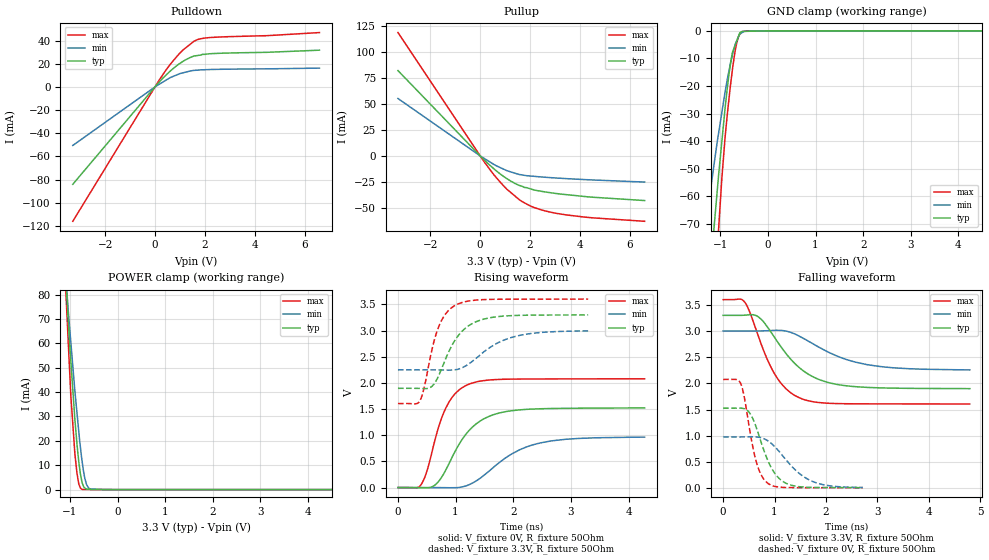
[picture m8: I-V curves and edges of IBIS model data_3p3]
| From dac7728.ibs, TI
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|   data_3p3 Model
[Model]   data_3p3
Model_type   I/O
Polarity   Non-Inverting
Enable   Active-Low
Vinl = 0.6
Vinh = 2.3
Vmeas = 1.65
Vref = 1.65
Cref = 10pF
Rref = 50
|   typ   min   max
|   (nom PVT)   (Fast PVT)   (slow PVT)
|C_comp from frequency method(F=50MHz)
|Average
C_comp   9.480e-12   7.960e-12   1.096e-11
|ON state : BUFFER OUTPUT TURNED HIGH
|C_comp   9.694e-12   8.160e-12   1.122e-11
|OFF state: BUFFER IN HIGH IMPEDANCE
|C_comp   9.266e-12   7.761e-12   1.070e-11
|C_comp from L-C Tank method(L=1nH)
|Average
|C_comp   8.7775e-12  7.5775e-12  9.971e-12
|ON state : BUFFER OUTPUT TURNED HIGH
|Resonant Frequency(Hz)   1.68e9   1.8e9   1.58e9
|C_comp   8.984e-12   7.826e-12   1.016e-11
|OFF state: BUFFER IN HIGH IMPEDANCE
|Resonant Frequency(Hz)   1.72e9   1.86e9   1.61e9
|C_comp   8.571e-12   7.329e-12   9.782e-12
| Where nom  PVT is Nominal Process,  3.3V,  33C
|   Fast PVT is Strong Process,   3.6V,  -40C
|   Slow PVT is Weak Process,   3V,  113C
[Voltage Range]   3.3   3   3.6
|Ambient Temperature   25   105   -40
|Junction Temperature
[Temperature Range]   33   113   -40
[Pullup Reference]   3.3   3   3.6
[Pulldown Reference]   0   0   0
[Power Clamp Reference]   3.3   3   3.6
[GND Clamp Reference]   0   0   0
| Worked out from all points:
|   slope of the pulldown table from 0 to 0.495 V, typ, clamps not added: 44 ohm
|   slope of the pullup table from 0 to 0.495 V, typ, clamps not added: 43.8 ohm
|   GND clamp passes 1 mA (typ) near -0.60 V on its own axis
|   POWER clamp passes 1 mA (typ) near -0.71 V on its own axis
|   falling waveform, V_fixture 3.3V, R_fixture 50Ohm: 20-80 % time 748ps typ, 999ps min, 546ps max; typ from 3.3 V to 1.9 V
|   rising waveform, V_fixture 0V, R_fixture 50Ohm: 20-80 % time 543ps typ, 776ps min, 372ps max; typ from 0 V to 1.52 V
|   rising waveform, V_fixture 3.3V, R_fixture 50Ohm: 20-80 % time 420ps typ, 633ps min, 286ps max; typ from 1.9 V to 3.3 V
|   falling waveform, V_fixture 0V, R_fixture 50Ohm: 20-80 % time 362ps typ, 577ps min, 246ps max; typ from 1.52 V to 0.006 V
[Pulldown]
|   Voltage   I(typ)   I(min)   I(max)
-3.3V     -84.11mA   -50.56mA   -116mA
18mV      443.3uA    274.6uA    641.4uA
273.6mV   6.576mA    3.631mA    9.304mA
633.6mV   14.12mA    8.199mA    20.06mA
939.6mV   19.39mA    10.93mA    27.83mA
1.247V    23.62mA    12.83mA    33.99mA
1.566V    26.63mA    14.23mA    39.43mA
1.814V    27.44mA    14.64mA    41.5mA
2.203V    28.63mA    14.99mA    42.59mA
4.5V      29.86mA    15.58mA    44.23mA
6.6V      31.7mA     16.21mA    46.9mA
[GND Clamp]
|   Voltage   I(typ)   I(min)   I(max)
-3.3V     -572.7mA   -387.4mA   -802.2mA
-1.361V   -118.9mA   -77.73mA   -170.9mA
-1.272V   -100mA     -65.91mA   -143mA
-1.184V   -81.73mA   -55mA      -115.6mA
-1.071V   -59.2mA    -40.91mA   -81.77mA
-1.036V   -52.29mA   -37.09mA   -71.86mA
-896.4mV  -27.44mA   -21.78mA   -37.88mA
-811.8mV  -14.96mA   -13.98mA   -23.71mA
-738mV    -7.483mA   -8.126mA   -12.99mA
-655.2mV  -3.679mA   -3.589mA   -4.387mA
-537.9mV  -215.9uA   -600.8uA   -323.7uA
6.6V      0A         0A         0A
[Pullup]
|   Voltage   I(typ)   I(min)   I(max)
-3.3V     82.34mA    55.4mA     119mA
172.8mV   -4.196mA   -2.62mA    -6.082mA
576mV     -13.01mA   -8.649mA   -18.98mA
939.6mV   -19.86mA   -12.81mA   -28.97mA
1.247V    -24.64mA   -15.61mA   -35.77mA
1.573V    -28.56mA   -17.98mA   -42.34mA
2.167V    -32.93mA   -19.76mA   -49.89mA
3.089V    -36.46mA   -21.42mA   -55.59mA
4.497V    -39.88mA   -23.24mA   -59.79mA
6.6V      -43.13mA   -25.28mA   -63.15mA
[POWER Clamp]
|   Voltage   I(typ)   I(min)   I(max)
-3.3V     869.3mA    734.6mA    1.044A
-1.084V   85.81mA    86.41mA    79.97mA
-1.032V   68.16mA    72.24mA    58.91mA
-982.8mV  52.97mA    60.65mA    38.83mA
-896.4mV  28.7mA     40.32mA    14.56mA
-853.2mV  18.73mA    31.56mA    6.771mA
-817.2mV  11.76mA    24.27mA    2.531mA
-756mV    3.952mA    13.19mA    210.4uA
-687mV    641.4uA    4.545mA    38.04uA
-651mV    146.4uA    2.075mA    32.51uA
-573mV    128.8uA    253uA      20.54uA
6.6V      0A         0A         0A
[Ramp]
R_load = 50
|   typ   min   max
dV/dt_r   0.915505/5.46681e-10   0.584669/7.93823e-10   1.24659/3.72445e-10
dV/dt_f   0.842302/7.50867e-10   0.450434/1.02002e-09   1.19671/5.45793e-10
[Falling Waveform]
V_fixture = 3.3V
V_fixture_min = 3V
V_fixture_max = 3.6V
R_fixture = 50Ohm
|   Time   V(typ)   V(min)   V(max)
0s        3.3V       3V         3.6V
420ps     3.304V     3V         3.552V
520ps     3.312V     3V         3.358V
680ps     3.275V     3.001V     2.917V
1ns       2.88V      3.013V     2.184V
1.24ns    2.549V     2.995V     1.882V
1.52ns    2.27V      2.882V     1.709V
2.02ns    2.023V     2.61V      1.62V
2.78ns    1.924V     2.362V     1.608V
4.8ns     1.899V     2.256V     1.606V
[Rising Waveform]
V_fixture = 0V
V_fixture_min = 0V
V_fixture_max = 0V
R_fixture = 50Ohm
|   Time   V(typ)   V(min)   V(max)
0s        2.468nV    3.31nV     2.196nV
400ps     -1.13mV    104.1uV    53.75mV
500ps     -5.322mV   191.2uV    305.5mV
620ps     30.96mV    120.7uV    815.2mV
820ps     315.3mV    -1.542mV   1.495V
1ns       708.6mV    -1.861mV   1.803V
1.22ns    1.073V     48.37mV    1.969V
1.64ns    1.386V     371mV      2.06V
2.36ns    1.501V     822.4mV    2.074V
4.28ns    1.522V     964.1mV    2.077V
[Rising Waveform]
V_fixture = 3.3V
V_fixture_min = 3V
V_fixture_max = 3.6V
R_fixture = 50Ohm
|   Time   V(typ)   V(min)   V(max)
0s        1.896V     2.249V     1.605V
380ps     1.894V     2.249V     1.658V
460ps     1.891V     2.249V     1.933V
580ps     1.924V     2.248V     2.585V
700ps     2.121V     2.247V     3.053V
820ps     2.439V     2.244V     3.308V
1ns       2.832V     2.252V     3.485V
1.36ns    3.17V      2.473V     3.582V
1.98ns    3.285V     2.87V      3.599V
3.3ns     3.298V     2.993V     3.6V
[Falling Waveform]
V_fixture = 0V
V_fixture_min = 0V
V_fixture_max = 0V
R_fixture = 50Ohm
|   Time   V(typ)   V(min)   V(max)
0s        1.525V     975.7mV    2.075V
340ps     1.526V     975.7mV    2.002V
400ps     1.518V     976.2mV    1.793V
500ps     1.453V     977.6mV    1.211V
640ps     1.172V     975.8mV    519.2mV
740ps     870.5mV    961.4mV    251.2mV
860ps     548mV      908mV      96.48mV
1.18ns    113.6mV    588.5mV    10.66mV
1.7ns     10.99mV    142.3mV    5.553mV
2.72ns    6.313mV    9.44mV     1.866mV
